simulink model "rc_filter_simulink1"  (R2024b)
settings: Solver=VariableStepAuto  StartTime=0.0  StopTime=10.0  RelTol=1e-3

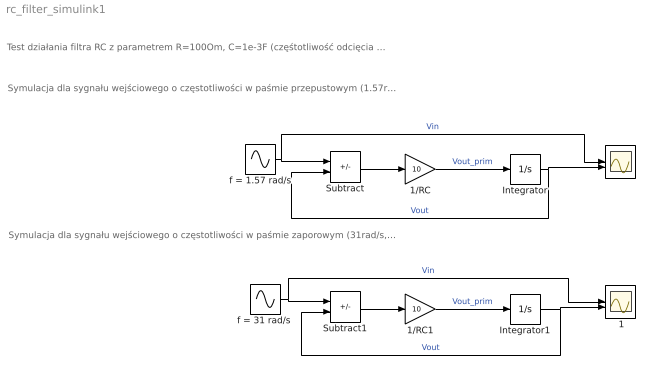
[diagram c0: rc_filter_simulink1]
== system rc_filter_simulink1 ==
  note: Symulacja dla sygnału wejściowego o częstotliwości w paśmie zaporowym (31rad/s, czyli ok. 5Hz)
  note: Test działania filtra RC z parametrem R=100Om, C=1e-3F (częśtotliwość odcięcia ok. 1.6Hz)
  note: Symulacja dla sygnału wejściowego o częstotliwości w paśmie przepustowym (1.57rad/s, czyli ok. 1/4Hz)
  " " : Scope  NumInputPorts=2
  " 1" : Scope  NumInputPorts=2
  1/RC : Gain  Gain=10
  1/RC1 : Gain  Gain=10
  Integrator : Integrator
  Integrator1 : Integrator
  Subtract : Sum  Inputs=+-
  Subtract1 : Sum  Inputs=+-
  f = 1.57 rad/s : Sin  Frequency=1.57  SampleTime=0
  "f = 31 rad/s " : Sin  Frequency=31  SampleTime=0
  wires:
  1/RC/1 -> Integrator/1  "Vout_prim"
  Integrator/1 -> Subtract/2, " "/2  "Vout"
  f = 1.57 rad/s/1 -> " "/1, Subtract/1  "Vin"
  Subtract/1 -> 1/RC/1
  "f = 31 rad/s "/1 -> Subtract1/1, " 1"/1  "Vin"
  Subtract1/1 -> 1/RC1/1
  1/RC1/1 -> Integrator1/1  "Vout_prim"
  Integrator1/1 -> Subtract1/2, " 1"/2  "Vout"
